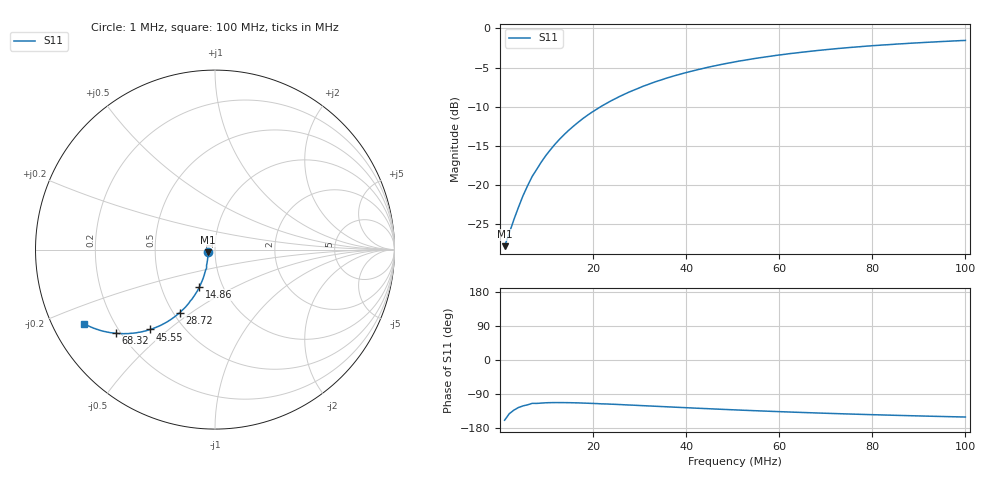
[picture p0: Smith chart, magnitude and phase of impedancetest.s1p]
# Hz S RI R 50.0
! written by SimSmith version 18.3b
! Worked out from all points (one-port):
!   101 points, 1 MHz to 100 MHz, reference 50 ohm
!   lowest |S11| = -27.8 dB at 1 MHz (marker M1), VSWR 1.08, Z = 46.3 - j1.36 ohm
!   |S11| at or under -10 dB: start of sweep to 21.62 MHz
!   S11 on the Smith chart (normalised r, x): 1 MHz: 0.93, -0.03; 14.86 MHz: 0.78, -0.34; 28.72 MHz: 0.54, -0.45; 45.55 MHz: 0.33, -0.43; 68.32 MHz: 0.18, -0.35; 100 MHz: 0.09, -0.26
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1000000  -0.038 -0.0146
1990000  -0.0387 -0.0303
2980000  -0.0405 -0.0444
3970000  -0.0418 -0.0587
4960000  -0.0442 -0.0733
5950000  -0.047 -0.0873
6940000  -0.047 -0.1035
8920000  -0.0565 -0.129
9910000  -0.0603 -0.1429
1.189e7  -0.0697 -0.1695
1.387e7  -0.0807 -0.195
1.486e7  -0.0865 -0.2076
1.783e7  -0.1069 -0.2436
1.981e7  -0.1216 -0.2661
2.278e7  -0.145 -0.2976
2.575e7  -0.1704 -0.3266
2.872e7  -0.1971 -0.352
3.367e7  -0.2449 -0.3887
3.862e7  -0.2929 -0.4168
4.555e7  -0.3602 -0.445
5.05e7  -0.4064 -0.4576
5.545e7  -0.4506 -0.4651
6.337e7  -0.5158 -0.468
6.832e7  -0.5536 -0.4662
7.525e7  -0.6006 -0.4597
8.02e7  -0.6313 -0.4526
8.812e7  -0.6747 -0.4385
1e8  -0.7295 -0.413
